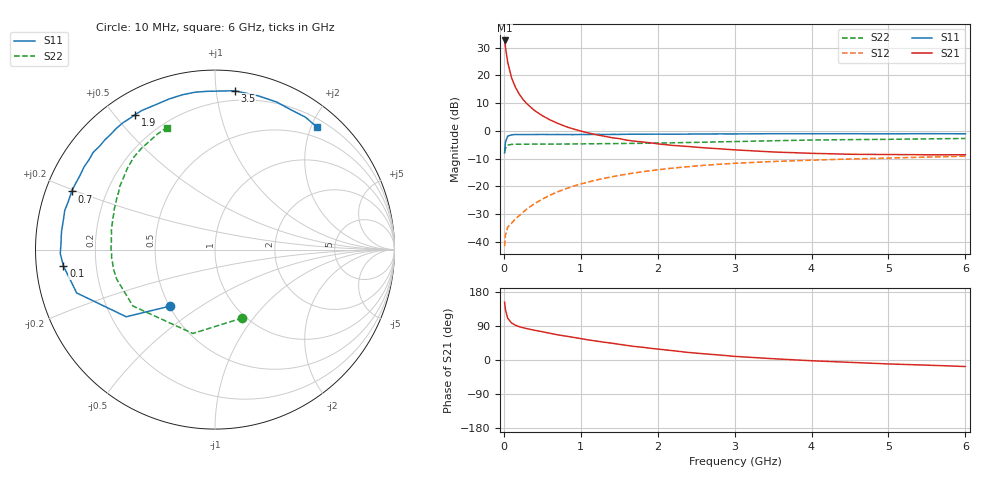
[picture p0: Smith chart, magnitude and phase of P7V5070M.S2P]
! SIEMENS Small Signal Semiconductors
! BFP196
! Si NPN RF Bipolar Junction Transistor in SOT143
! VCE = 0.5 V  IC = 70 mA
! Common Emitter S-Parameters:  May  1996
# GHz  S  MA  R  50
!  f  S11  S21  S12  S22
! GHz  MAG  ANG  MAG  ANG  MAG  ANG  MAG  ANG
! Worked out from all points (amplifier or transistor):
!   36 points, 10 MHz to 6 GHz, reference 50 ohm
!   highest |S21| = 32.6 dB at 10 MHz (marker M1)
!   |S21| within 3 dB of that: start of sweep to 24.2 MHz
!   unconditionally stable (mu >= 1): start of sweep to 10.92 MHz; 180.9 MHz to end of sweep
!   at 250 MHz: K = 1.13, MAG = 18.1 dB, |S12| = -29.3 dB
!   at 1.4 GHz: K = 1.25, MAG = 4.1 dB, |S12| = -16.5 dB
!   at 6 GHz: K = 1.08, MAG = -1.5 dB, |S12| = -9.1 dB
!   S11 on the Smith chart (normalised r, x): 10 MHz: 0.50, -0.38; 100 MHz: 0.08, -0.05; 700 MHz: 0.08, +0.19; 1.9 GHz: 0.09, +0.57; 3.5 GHz: 0.13, +1.12; 6 GHz: 0.32, +2.08
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0.01  0.4032 -128.6  42.62 152.7  0.0084 58.4  0.4104 -68.2
0.02  0.6202 -142.9  33.02 134.0  0.0132 47.7  0.4833 -104.8
0.05  0.8076 -162.6  17.34 110.1  0.0185 36.0  0.555 -145.5
0.1  0.8498 -173.9  9.082 97.7  0.0217 39.5  0.5719 -163.3
0.15  0.8624 -178.6  6.143 91.9  0.026 45.7  0.5765 -169.6
0.2  0.8586 177.8  4.619 87.9  0.0297 51.5  0.5755 -173.2
0.25  0.8599 175.1  3.684 85.1  0.0343 54.4  0.5781 -175.7
0.3  0.8609 173.1  3.082 82.8  0.0393 57.0  0.5763 -177.3
0.4  0.861 168.4  2.33 78.4  0.0492 60.7  0.5786 -179.8
0.5  0.8651 165.4  1.882 74.7  0.059 61.9  0.5791 178.1
0.6  0.8601 161.7  1.58 70.5  0.0697 62.3  0.5786 176.4
0.7  0.8618 157.9  1.37 66.4  0.08 62.2  0.5797 174.9
0.9  0.858 151.4  1.089 59.9  0.1008 60.1  0.5822 172.1
1.1  0.8623 144.5  0.918 52.9  0.1204 57.7  0.5872 169.4
1.6  0.8708 129.1  0.681 38.5  0.1668 49.6  0.5954 162.8
1.9  0.8735 120.5  0.612 31.1  0.1916 44.4  0.6026 158.9
2.2  0.8722 112.4  0.548 24.5  0.2142 39.3  0.6106 154.8
2.8  0.884 97.1  0.477 13.2  0.251 29.3  0.6367 146.5
3.5  0.8916 83.0  0.418 3.4  0.2814 18.5  0.6652 137.4
4.5  0.8911 67.3  0.38 -6.2  0.3122 6.0  0.6975 125.8
5.5  0.8934 55.6  0.372 -13.6  0.338 -4.6  0.7195 116.4
6  0.8882 50.4  0.372 -17.2  0.3502 -10.4  0.7311 111.5
